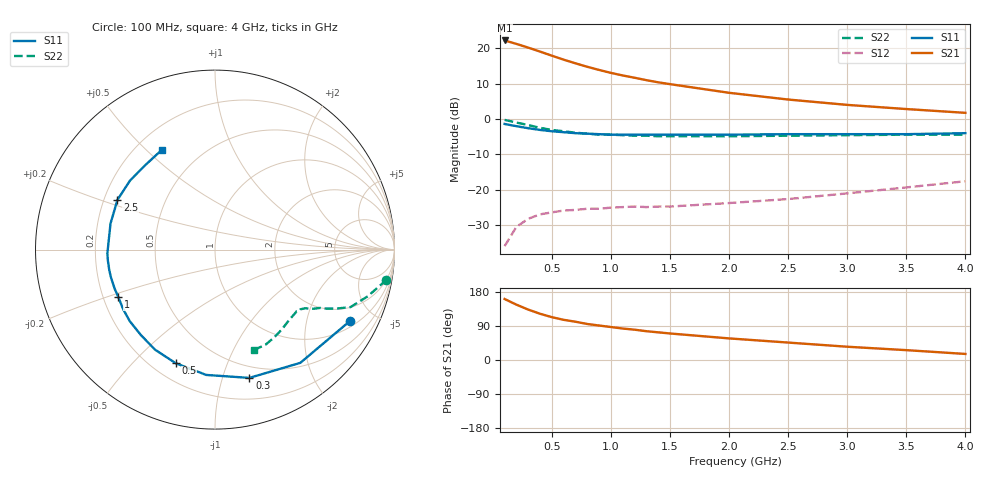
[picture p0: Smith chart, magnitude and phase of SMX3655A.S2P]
! HSMX-3655 Common Emitter
! Vce=10V Ic=5ma
# ghz s ma r 50
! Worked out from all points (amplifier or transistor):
!   20 points, 100 MHz to 4 GHz, reference 50 ohm
!   highest |S21| = 22.2 dB at 100 MHz (marker M1)
!   |S21| within 3 dB of that: start of sweep to 386.8 MHz
!   unconditionally stable (mu >= 1): 1.473 GHz to 3.775 GHz
!   at 400 MHz: K = 0.32, MSG = 23.0 dB, |S12| = -26.9 dB
!   at 1.1 GHz: K = 0.78, MSG = 18.6 dB, |S12| = -24.9 dB
!   at 4 GHz: K = 0.94, MSG = 9.7 dB, |S12| = -17.6 dB
!   S11 on the Smith chart (normalised r, x): 100 MHz: 1.25, -3.60; 300 MHz: 0.39, -1.23; 500 MHz: 0.29, -0.67; 1 GHz: 0.26, -0.22; 2.5 GHz: 0.26, +0.23; 4 GHz: 0.30, +0.56
0.1  0.85 -28.0  12.83 161.0  0.016 71.0  0.97 -10.0
0.2  0.79 -53.0  11.47 146.0  0.03 63.0  0.89 -17.0
0.3  0.74 -75.0  10.16 133.0  0.039 53.0  0.82 -23.0
0.4  0.7 -94.0  8.93 122.0  0.045 46.0  0.75 -26.0
0.5  0.67 -109.0  7.82 113.0  0.048 41.0  0.7 -28.0
0.6  0.65 -121.0  6.87 106.0  0.051 39.0  0.67 -29.0
0.7  0.63 -131.0  6.1 101.0  0.052 37.0  0.64 -31.0
0.8  0.62 -140.0  5.45 95.0  0.054 37.0  0.62 -32.0
0.9  0.61 -147.0  4.92 91.0  0.054 35.0  0.6 -33.0
1  0.6 -154.0  4.47 87.0  0.056 35.0  0.6 -33.0
1.1  0.6 -159.0  4.11 83.0  0.057 35.0  0.59 -34.0
1.2  0.6 -165.0  3.82 80.0  0.058 36.0  0.58 -35.0
1.3  0.6 -169.0  3.53 76.0  0.057 36.0  0.58 -36.0
1.4  0.6 -174.0  3.29 73.0  0.058 37.0  0.57 -37.0
1.5  0.6 -178.0  3.1 70.0  0.058 38.0  0.57 -38.0
2  0.6 166.0  2.34 57.0  0.065 46.0  0.57 -44.0
2.5  0.61 153.0  1.88 46.0  0.074 53.0  0.58 -50.0
3  0.61 141.0  1.58 35.0  0.089 57.0  0.59 -56.0
3.5  0.61 130.0  1.38 26.0  0.108 61.0  0.6 -62.0
4  0.63 118.0  1.22 16.0  0.132 60.0  0.6 -69.0
